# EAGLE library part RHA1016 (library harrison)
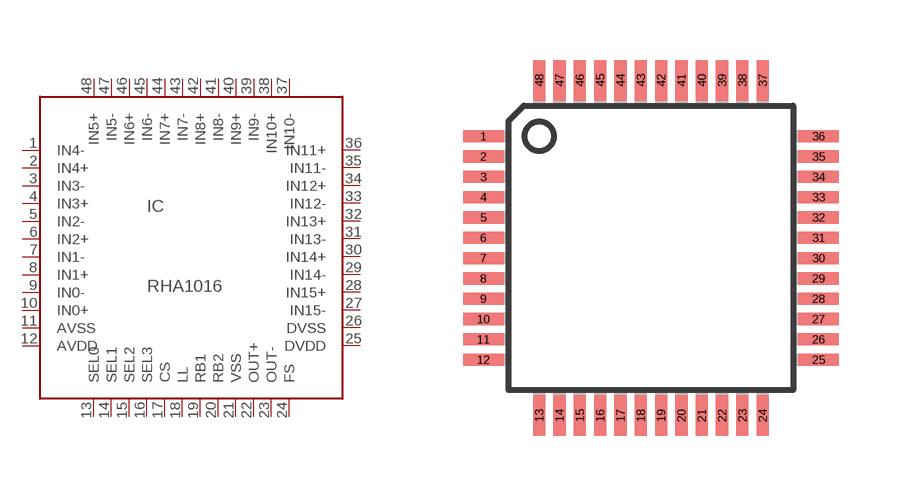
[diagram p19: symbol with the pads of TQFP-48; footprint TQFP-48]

Designator prefix IC

## RHA1016QFP  [TQFP-48]
1  IN4-
2  IN4+
3  IN3-
4  IN3+
5  IN2-
6  IN2+
7  IN1-
8  IN1+
9  IN0-
10  IN0+
11  AVSS
12  AVDD
13  SEL0
14  SEL1
15  SEL2
16  SEL3
17  CS
18  LL
19  RB1
20  RB2
21  VSS
22  OUT+
23  OUT-
24  FS
25  DVDD
26  DVSS
27  IN15-
28  IN15+
29  IN14-
30  IN14+
31  IN13-
32  IN13+
33  IN12-
34  IN12+
35  IN11-
36  IN11+
37  IN10-
38  IN10+
39  IN9-
40  IN9+
41  IN8-
42  IN8+
43  IN7-
44  IN7+
45  IN6-
46  IN6+
47  IN5-
48  IN5+

## Footprint TQFP-48 (pad centres in mm)
smd 1.016 x 0.305: 1 -4.191,2.794; 2 -4.191,2.286; 3 -4.191,1.778; 4 -4.191,1.27; 5 -4.191,0.762; 6 -4.191,0.254; 7 -4.191,-0.254; 8 -4.191,-0.762; 9 -4.191,-1.27; 10 -4.191,-1.778; 11 -4.191,-2.286; 12 -4.191,-2.794; 25 4.191,-2.794; 26 4.191,-2.286; 27 4.191,-1.778; 28 4.191,-1.27; 29 4.191,-0.762; 30 4.191,-0.254; 31 4.191,0.254; 32 4.191,0.762; 33 4.191,1.27; 34 4.191,1.778; 35 4.191,2.286; 36 4.191,2.794
smd 0.305 x 1.016: 13 -2.794,-4.191; 14 -2.286,-4.191; 15 -1.778,-4.191; 16 -1.27,-4.191; 17 -0.762,-4.191; 18 -0.254,-4.191; 19 0.254,-4.191; 20 0.762,-4.191; 21 1.27,-4.191; 22 1.778,-4.191; 23 2.286,-4.191; 24 2.794,-4.191; 37 2.794,4.191; 38 2.286,4.191; 39 1.778,4.191; 40 1.27,4.191; 41 0.762,4.191; 42 0.254,4.191; 43 -0.254,4.191; 44 -0.762,4.191; 45 -1.27,4.191; 46 -1.778,4.191; 47 -2.286,4.191; 48 -2.794,4.191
